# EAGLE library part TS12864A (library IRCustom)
KS0108 based display. Some have slightly different pinouts so double check!
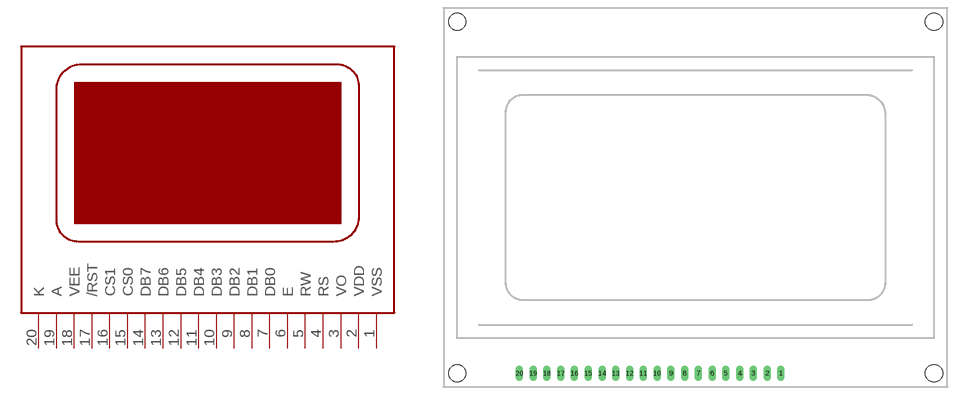
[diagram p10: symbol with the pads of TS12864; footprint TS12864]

Designator prefix -

## TS12864A  [TS12864]
1  VSS  sup
2  VDD  sup
3  VO  in
4  RS  in
5  RW  in
6  E  in
7  DB0
8  DB1
9  DB2
10  DB3
11  DB4
12  DB5
13  DB6
14  DB7
15  CS0  in
16  CS1  in
17  /RST  in
18  VEE  sup
19  A  sup
20  K  in

## Footprint TS12864 (pad centres in mm)
drill 0.9 long: 1 48.26,0; 2 45.72,0; 3 43.18,0; 4 40.64,0; 5 38.1,0; 6 35.56,0; 7 33.02,0; 8 30.48,0; 9 27.94,0; 10 25.4,0; 11 22.86,0; 12 20.32,0; 13 17.78,0; 14 15.24,0; 15 12.7,0; 16 10.16,0; 17 7.62,0; 18 5.08,0; 19 2.54,0; 20 0,0
hole 3.2 at -11.5,65
hole 3.2 at 76.5,65
hole 3.2 at -11.5,0
hole 3.2 at 76.5,0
